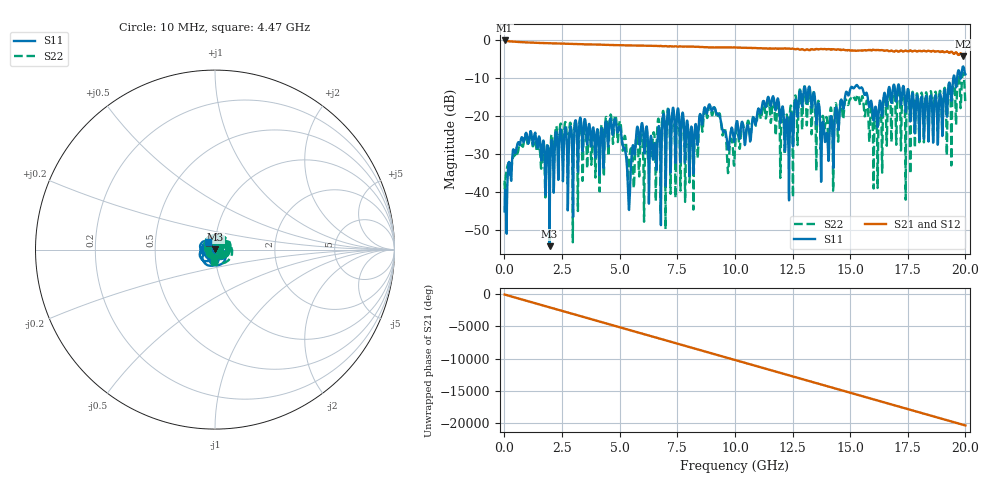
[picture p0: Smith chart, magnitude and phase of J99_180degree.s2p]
!Keysight Technologies,N5222A,MY51421036,A.10.65.16
!Date: Friday, March 31, 2023 15:05:10
!Correction: S11(Full 2 Port(1,2))
!S21(Full 2 Port(1,2))
!S12(Full 2 Port(1,2))
!S22(Full 2 Port(1,2))
!S2P File: Measurements: S11, S21, S12, S22:
# Hz S  dB  R 50
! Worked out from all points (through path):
!   2000 points, 10 MHz to 20 GHz, reference 50 ohm
!   highest |S21| = -0.04 dB at 10 MHz (marker M1); lowest = -4.2 dB at 19.9 GHz (marker M2)
!   group delay of S21, straight-line fit = 2.84 ns
!   lowest |S11| = -54.1 dB at 1.96 GHz (marker M3), VSWR 1.00, Z = 50.1 + j0.169 ohm
!   |S11| at or under -10 dB: start of sweep to 19.48 GHz; 19.54 GHz to 19.64 GHz (100.7 MHz wide, 0.514 % of centre); 19.78454 GHz to 19.7975 GHz (12.96 MHz wide, 0.0655 % of centre)
!   |S22| runs from -53.1 to -8.5 dB; largest |S21 - S12| = 0.022
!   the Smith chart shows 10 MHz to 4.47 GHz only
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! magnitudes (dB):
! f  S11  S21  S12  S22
! 10 MHz  -45.0  0.0  -0.1  -36.9
! 680 MHz  -27.3  -0.5  -0.4  -27.5
! 1.96 GHz  -54.1  -0.8  -0.7  -40.6
! 3.35 GHz  -23.5  -1.0  -1.0  -24.7
! 4.88 GHz  -23.5  -1.3  -1.2  -23.3
! 5.4 GHz  -44.5  -1.3  -1.3  -33.1
! 5.83 GHz  -25.3  -1.4  -1.4  -33.9
! 6.68 GHz  -23.2  -1.5  -1.5  -20.6
! 7.56 GHz  -18.9  -1.6  -1.6  -19.9
! 8.12 GHz  -22.8  -1.7  -1.7  -24.3
! 8.96 GHz  -18.0  -1.8  -1.8  -18.1
! 10.01 GHz  -24.3  -1.9  -1.9  -28.4
! 11.61 GHz  -15.7  -2.2  -2.2  -18.0
! 12.27 GHz  -20.3  -2.2  -2.2  -20.1
! 13.34 GHz  -17.7  -2.3  -2.3  -22.4
! 14 GHz  -24.8  -2.4  -2.3  -21.0
! 15.09 GHz  -12.3  -2.7  -2.7  -15.3
! 16.1 GHz  -17.5  -2.6  -2.5  -18.0
! 16.67 GHz  -12.7  -2.8  -2.8  -13.2
! 18.9 GHz  -14.0  -3.1  -2.9  -13.3
! 19.9 GHz  -6.9  -4.2  -3.9  -8.5
! 20 GHz  -9.0  -3.6  -3.4  -16.3
